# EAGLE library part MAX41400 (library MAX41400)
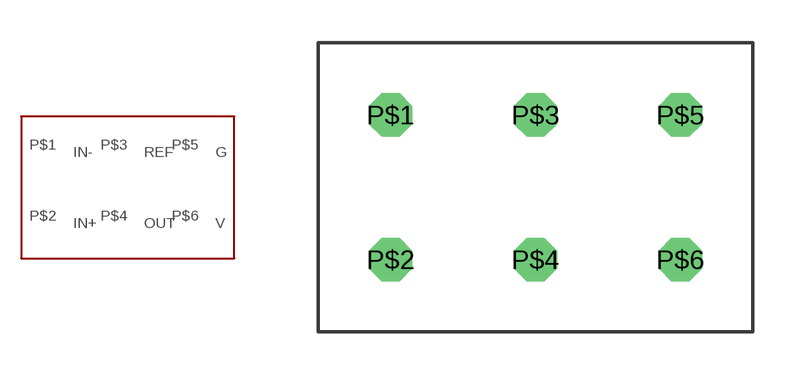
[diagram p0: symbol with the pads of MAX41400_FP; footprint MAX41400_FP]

Designator prefix -

## MAX41400  [MAX41400_FP]
P$1  IN-
P$2  IN+
P$3  REF
P$4  OUT
P$5  G
P$6  V

## Footprint MAX41400_FP (pad centres in mm)
drill 1.016 octagon: P$1 -5.08,5.08; P$2 -5.08,0; P$3 0,5.08; P$4 0,0; P$5 5.08,5.08; P$6 5.08,0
